(* Logix 5000 AddOnInstructionDefinition export Banner_K50ProTouch_Param_v4; software revision 33.00 *)

TYPE Banner_IOL_Port_v4 :   // UDT that has all of the data items necessary to communicate with a specific Port on a IO-Link Master
STRUCT
   Port_Controlled : INT;   // Each bit represents a port on an IO-Link Master. Set to 1 to tell AOI to control that port.
   Port_Activate : INT;   // Each bit represents a port on an IO-Link Master. When ON that port will process any commands in queue.
   Port_Read : INT;   // Each bit represents a port on an IO-Link Master. Used to determine when device AOI has requested a Read command.
   Port_Write : INT;   // Each bit represents a port on an IO-Link Master. Used to determine when device AOI has requested a Write command.
   Port_RW_Complete : INT;   // Each bit represents a port on an IO-Link Master. Tells device AOI that Read or Write request has been completed.
   Port_Device_Read : INT;
   Data_Transfer : SINT[190];   // Array to transfer data from IO-Master to device AOIs.
END_STRUCT
END_TYPE

TYPE Banner_K50ProTouch_RD_v4 :   // UDT with all of the Read only parameters for K50 Pro Touch.
STRUCT
   Master_Cycle_Time : INT;
   Min_Cycle_Time : INT;
   M_Sequence_Capability : INT;
   IO_Link_Version_ID : INT;
   Process_Data_Input_Length : INT;
   Process_Data_Output_Length : INT;
   Combined_Vendor_ID : DINT;   // IO-Link Vendor ID
   Vendor_ID1 : INT;
   Vendor_ID2 : INT;
   Combined_Device_ID : DINT;   // IO-Link Device ID
   Device_ID1 : INT;
   Device_ID2 : INT;
   Device_ID3 : INT;
   Serial_Number : STRING;
END_STRUCT
END_TYPE

TYPE Banner_K50ProTouch_SP_v4 :   // UDT for K50 Pro Touch with the State Parameters structure.
STRUCT
   Type : SINT;   // 0 = Off, 1 = Steady, 2 = Flash, 3 = Two Color Flash, 4 = 50/50, 5 = 50/50 Rotate, 6 = Chase, 7 = Intensity Sweep, 8 = Sequence.
   Direction : SINT;   // 0 = CCW, 1 = CW.
   Pattern : SINT;   // 0 = Flash, 1 = Strobe, 2 = Three Pulse, 3 = SOS, 4 = Random.
   Speed : SINT;   // 0 = Slow, 1 = Medium, 2 = Fast, 3 = Custom.
   Vibration_Feedback : SINT;   // 0 = Off, 1 = On, 2 = Pattern. Not available in all models.
   Off_Delay_Type : SINT;   // 0 =Leading Edge, 1 = Trailing Edge.
   Off_Delay : DINT;   // 0 to 65535 in ms. Length of time before the device returns to 'touch inactive' state after button is released.
   Static_Sequence : INT;   // 0 to 255. Value describing the LED position of the device.
   Sequence_Start_Location : SINT;   // 0 = LED1, 1 = LED2, 2 = LED3, 3 = LED4, 4 = LED5, 5 = LED6, 6 = LED7, 7 = LED8.
   Color_1 : SINT;   // 0 = Green, 1 = Red, 2 = Orange, 3 = Amber, 4 = Yellow, 5 = Lime Green, 6 = Spring Green, 7 = Cyan, 8 = SKy Blue, 9 = Blue, 10 = Violet, 11 = Magenta, 12 = Rose, 13 = White, 14 Custom 1, 15 = Custom 2.
   Color_1_Intensity : SINT;   // 0 = High, 1 = Medium, 2 = Low, 3 = Off, 4 = Custom.
   Color_2 : SINT;   // 0 = Green, 1 = Red, 2 = Orange, 3 = Amber, 4 = Yellow, 5 = Lime Green, 6 = Spring Green, 7 = Cyan, 8 = SKy Blue, 9 = Blue, 10 = Violet, 11 = Magenta, 12 = Rose, 13 = White, 14 Custom 1, 15 = Custom 2.
   Color_2_Intensity : SINT;   // 0 = High, 1 = Medium, 2 = Low, 3 = Off, 4 = Custom.
END_STRUCT
END_TYPE

TYPE Banner_K50ProTouch_v4 :   // UDT with all of the parameters for K50 Pro Touch.
STRUCT
   Initial_Global_Read : BOOL;   // Determines if all of the IO-Link data has been read into the PLC yet
   Command : INT;   // Value placed in here will activate a read or write to a specifc IO-Link Index
   Read_Data : Banner_K50ProTouch_RD_v4;   // All read data
   Write_Data : Banner_K50ProTouch_WD_v4;   // All data that can be written to.
   Archive : Banner_K50ProTouch_WD_v4;   // Archive of the write data.
   Reset : BOOL;
END_STRUCT
END_TYPE

TYPE Banner_K50ProTouch_WD_v4 :   // UDT that stores the Write Data for a K50 Pro Touch.
STRUCT
   System_Command : INT;   // See IODD file for list of commands that can be activated via the System Command interface
   Parameter_Access_Lock : SINT;   // Write access to all read/write parameters is block when this bit is ON.
   Data_Storage_Lock : SINT;   // Data storage mechanism is inhibited when bit is ON.
   Local_Parameterization_Lock : SINT;   // Parameteriation via local control elementes is inhibited.
   Local_User_Interface_Lock : SINT;   // Operation of the hmi on the device is disabled.
   Operation_Mode : SINT;   // 0 = Multicolor, 1 = Four State Full Logic, 2 = Advanced, 3 = LED Control, 4 = Demo.
   Custom_Intensity : SINT;   // 0 to 100 %
   Custom_Flash_Rate : INT;   // Range 5 to 200 (.5 to 20 converted rate).
   Restrict_to_Gamut : SINT;   // 0 = Off, 1 = On.
   Touch_Sensitivity : SINT;   // 0 = Low, 1 = High.
   Function : SINT;   // 0 = Momentary, 1 = Latched.
   Mute_Enable : SINT;   // 0 = Off, 1 = On.
   On_Delay : DINT;   // 0 to 65535 in ms. Length of time the touch button needs to be pressed to trigger touch active state.
   Output_State : SINT;   // 0 = NO, 1 = NC.
   Off_Delay_Type : SINT;   // 0 = Leading Edge, 1 = Trailing Edge.
   Off_Delay : DINT;   // 0 to 65535 in ms. Length of time before the device returns to the 'touch inactive' state after button is released.
   State_Parameters : Banner_K50ProTouch_SP_v4[5];   // State Parameters. 1 through 4 will have values.
   CC1_Red : INT;   // 0-255. Custom 1 Red.
   CC1_Green : INT;   // 0-255. Custom 1 Green.
   CC1_Blue : INT;   // 0-255. Custom 1 Blue.
   CC2_Red : INT;   // 0-255. Custom 2 Red.
   CC2_Green : INT;   // 0-255. Custom 2 Green.
   CC_Blue : INT;   // 0-255. Custom 2 Blue.
END_STRUCT
END_TYPE

ADD_ON_INSTRUCTION Banner_K50ProTouch_Param_v4   (* revision 4.2, vendor Banner Engineering *)
// AOI to read and write parameter data to an IO-Link K50 Pro Touch.
// Revision note:
// Write operation for Index 82 and 83 had wrong size. Changed szie to value of 3.
VAR_IN_OUT
   K50ProTouch : Banner_K50ProTouch_v4; {required}
   Port_Data : Banner_IOL_Port_v4; {required}
END_VAR
VAR_INPUT
   Port : DINT; {required}
END_VAR
VAR
   Local_Control : DINT; {access None}
   Global_Read_Command_Value : INT; {access None}
   Global_Write_Command_Value : INT; {access None}
   Command_Being_Processed : BOOL; {access None}
   Update_Archive : BOOL; {access None}
   Index_Write_Control : DINT; {access None}
   Index_Write_Inprocess : INT; {access None}
   Temp_Excess_Gain : DINT[2]; {access None}
   Inprocess_Index : DINT; {access None}
   SP_Index : DINT; {access None}   // State Parameters Index
   SP_Write_Index : DINT; {access None}
   SP_R_Index : DINT; {access None}
   SP_W_Index : DINT; {access None}
END_VAR

ROUTINE Logic   (* ladder *)
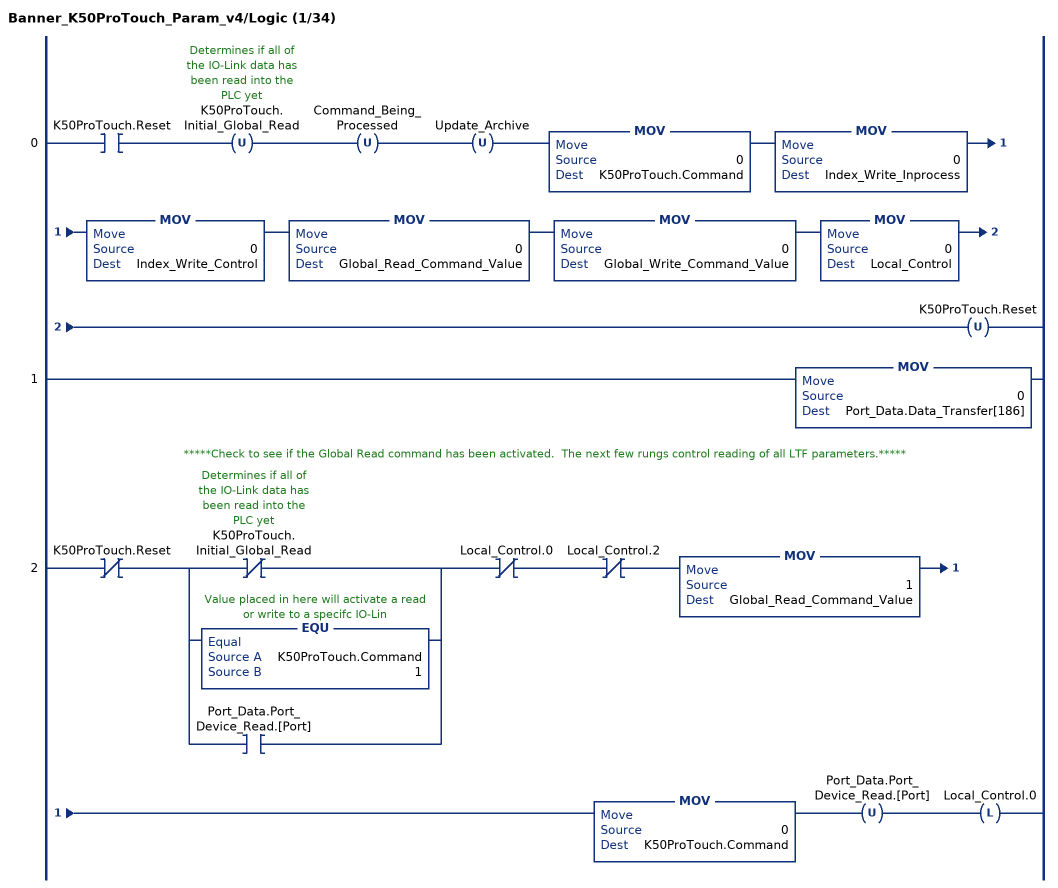
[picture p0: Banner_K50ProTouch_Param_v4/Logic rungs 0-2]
   0: XIC(K50ProTouch.Reset)OTU(K50ProTouch.Initial_Global_Read)OTU(Command_Being_Processed)OTU(Update_Archive)MOV(0,K50ProTouch.Command)MOV(0,Index_Write_Inprocess)MOV(0,Index_Write_Control)MOV(0,Global_Read_Command_Value)MOV(0,Global_Write_Command_Value)MOV(0,Local_Control)OTU(K50ProTouch.Reset);
   1: MOV(0,Port_Data.Data_Transfer[186]);
   // *****Check to see if the Global Read command has been activated.  The next few rungs control reading of all LTF parameters.*****
   2: XIO(K50ProTouch.Reset)[XIO(K50ProTouch.Initial_Global_Read) ,EQU(K50ProTouch.Command,1) ,XIC(Port_Data.Port_Device_Read.[Port]) ]XIO(Local_Control.0)XIO(Local_Control.2)MOV(1,Global_Read_Command_Value)MOV(0,K50ProTouch.Command)OTU(Port_Data.Port_Device_Read.[Port])OTL(Local_Control.0);
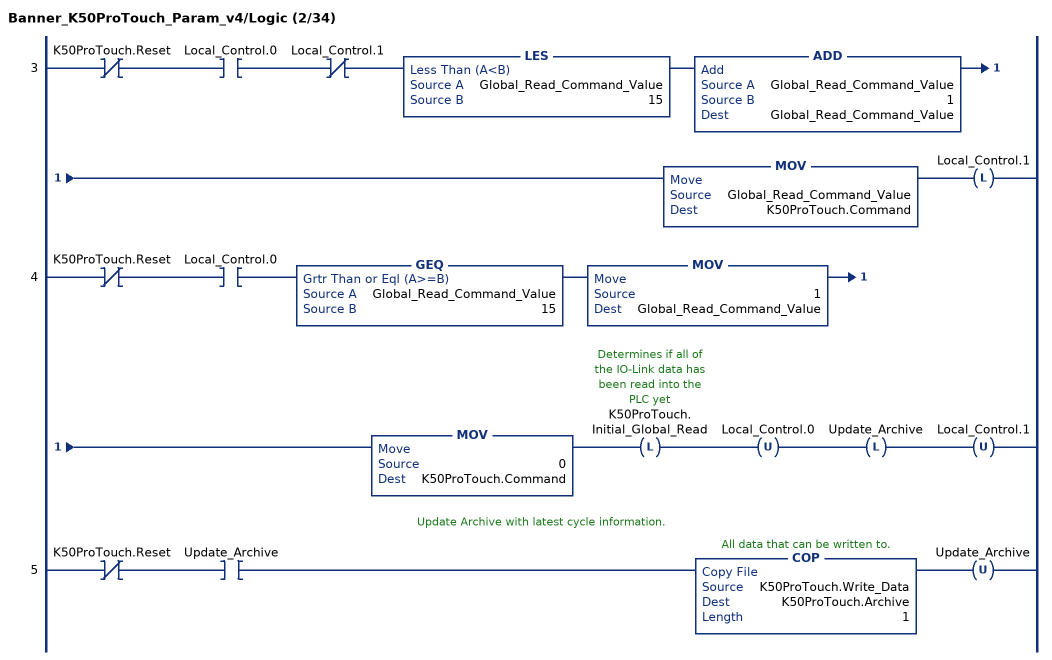
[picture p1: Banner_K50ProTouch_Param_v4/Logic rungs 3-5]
   3: XIO(K50ProTouch.Reset)XIC(Local_Control.0)XIO(Local_Control.1)LES(Global_Read_Command_Value,15)ADD(Global_Read_Command_Value,1,Global_Read_Command_Value)MOV(Global_Read_Command_Value,K50ProTouch.Command)OTL(Local_Control.1);
   4: XIO(K50ProTouch.Reset)XIC(Local_Control.0)GEQ(Global_Read_Command_Value,15)MOV(1,Global_Read_Command_Value)MOV(0,K50ProTouch.Command)OTL(K50ProTouch.Initial_Global_Read)OTU(Local_Control.0)OTL(Update_Archive)OTU(Local_Control.1);
   // Update Archive with latest cycle information.
   5: XIO(K50ProTouch.Reset)XIC(Update_Archive)COP(K50ProTouch.Write_Data,K50ProTouch.Archive,1)OTU(Update_Archive);
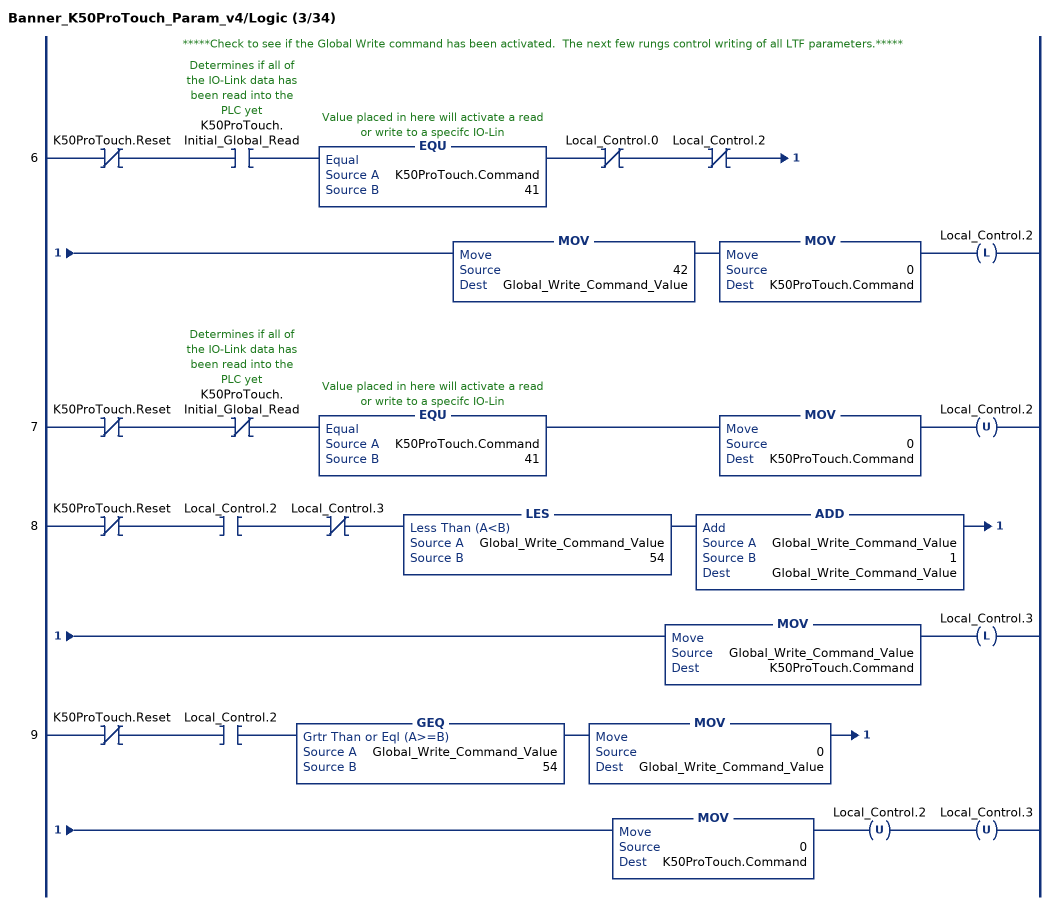
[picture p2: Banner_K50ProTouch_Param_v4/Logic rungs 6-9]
   // *****Check to see if the Global Write command has been activated.  The next few rungs control writing of all LTF parameters.*****
   6: XIO(K50ProTouch.Reset)XIC(K50ProTouch.Initial_Global_Read)EQU(K50ProTouch.Command,41)XIO(Local_Control.0)XIO(Local_Control.2)MOV(42,Global_Write_Command_Value)MOV(0,K50ProTouch.Command)OTL(Local_Control.2);
   7: XIO(K50ProTouch.Reset)XIO(K50ProTouch.Initial_Global_Read)EQU(K50ProTouch.Command,41)MOV(0,K50ProTouch.Command)OTU(Local_Control.2);
   8: XIO(K50ProTouch.Reset)XIC(Local_Control.2)XIO(Local_Control.3)LES(Global_Write_Command_Value,54)ADD(Global_Write_Command_Value,1,Global_Write_Command_Value)MOV(Global_Write_Command_Value,K50ProTouch.Command)OTL(Local_Control.3);
   9: XIO(K50ProTouch.Reset)XIC(Local_Control.2)GEQ(Global_Write_Command_Value,54)MOV(0,Global_Write_Command_Value)MOV(0,K50ProTouch.Command)OTU(Local_Control.2)OTU(Local_Control.3);
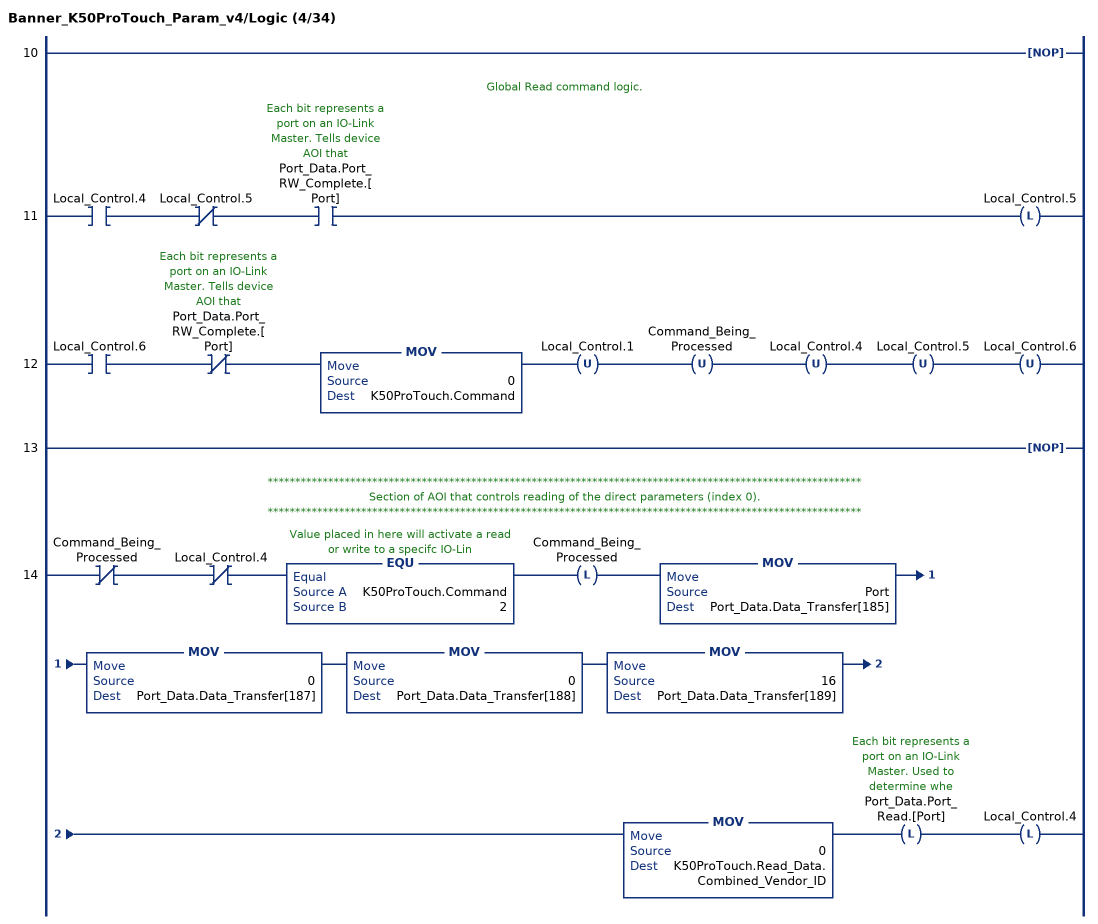
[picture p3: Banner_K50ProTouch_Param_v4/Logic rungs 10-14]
   10: NOP();
   // Global Read command logic.
   11: XIC(Local_Control.4)XIO(Local_Control.5)XIC(Port_Data.Port_RW_Complete.[Port])OTL(Local_Control.5);
   12: XIC(Local_Control.6)XIO(Port_Data.Port_RW_Complete.[Port])MOV(0,K50ProTouch.Command)OTU(Local_Control.1)OTU(Command_Being_Processed)OTU(Local_Control.4)OTU(Local_Control.5)OTU(Local_Control.6);
   13: NOP();
   // ************************************************************************************************************
   // Section of AOI that controls reading of the direct parameters (index 0).
   // ************************************************************************************************************
   14: XIO(Command_Being_Processed)XIO(Local_Control.4)EQU(K50ProTouch.Command,2)OTL(Command_Being_Processed)MOV(Port,Port_Data.Data_Transfer[185])MOV(0,Port_Data.Data_Transfer[187])MOV(0,Port_Data.Data_Transfer[188])MOV(16,Port_Data.Data_Transfer[189])MOV(0,K50ProTouch.Read_Data.Combined_Vendor_ID)OTL(Port_Data.Port_Read.[Port])OTL(Local_Control.4);
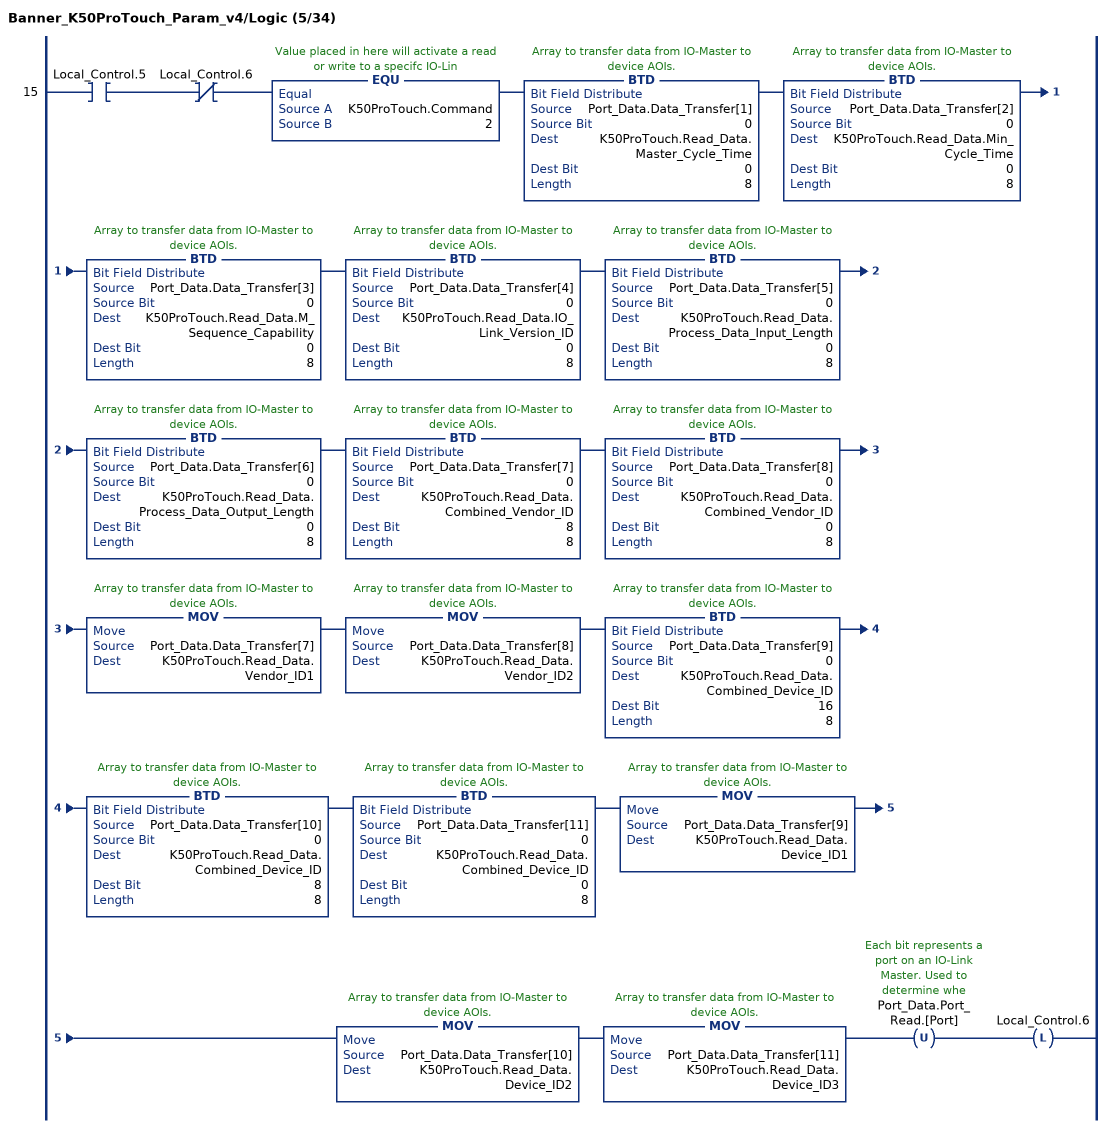
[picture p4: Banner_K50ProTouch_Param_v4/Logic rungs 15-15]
   15: XIC(Local_Control.5)XIO(Local_Control.6)EQU(K50ProTouch.Command,2)BTD(Port_Data.Data_Transfer[1],0,K50ProTouch.Read_Data.Master_Cycle_Time,0,8)BTD(Port_Data.Data_Transfer[2],0,K50ProTouch.Read_Data.Min_Cycle_Time,0,8)BTD(Port_Data.Data_Transfer[3],0,K50ProTouch.Read_Data.M_Sequence_Capability,0,8)BTD(Port_Data.Data_Transfer[4],0,K50ProTouch.Read_Data.IO_Link_Version_ID,0,8)BTD(Port_Data.Data_Transfer[5],0,K50ProTouch.Read_Data.Process_Data_Input_Length,0,8)BTD(Port_Data.Data_Transfer[6],0,K50ProTouch.Read_Data.Process_Data_Output_Length,0,8)BTD(Port_Data.Data_Transfer[7],0,K50ProTouch.Read_Data.Combined_Vendor_ID,8,8)BTD(Port_Data.Data_Transfer[8],0,K50ProTouch.Read_Data.Combined_Vendor_ID,0,8)MOV(Port_Data.Data_Transfer[7],K50ProTouch.Read_Data.Vendor_ID1)MOV(Port_Data.Data_Transfer[8],K50ProTouch.Read_Data.Vendor_ID2)BTD(Port_Data.Data_Transfer[9],0,K50ProTouch.Read_Data.Combined_Device_ID,16,8)BTD(Port_Data.Data_Transfer[10],0,K50ProTouch.Read_Data.Combined_Device_ID,8,8)BTD(Port_Data.Data_Transfer[11],0,K50ProTouch.Read_Data.Combined_Device_ID,0,8)MOV(Port_Data.Data_Transfer[9],K50ProTouch.Read_Data.Device_ID1)MOV(Port_Data.Data_Transfer[10],K50ProTouch.Read_Data.Device_ID2)MOV(Port_Data.Data_Transfer[11],K50ProTouch.Read_Data.Device_ID3)OTU(Port_Data.Port_Read.[Port])OTL(Local_Control.6);
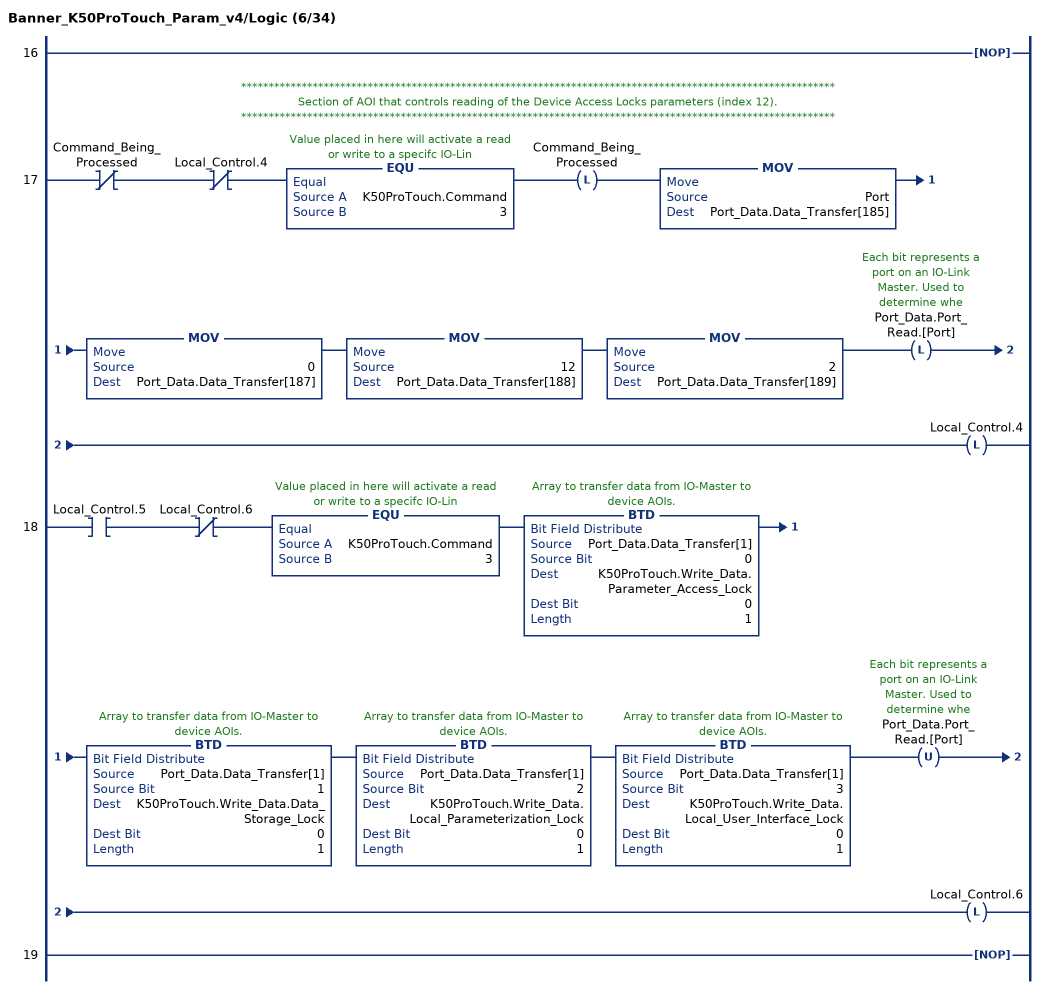
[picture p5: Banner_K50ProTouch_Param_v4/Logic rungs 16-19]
   16: NOP();
   // ************************************************************************************************************
   // Section of AOI that controls reading of the Device Access Locks parameters (index 12).
   // ************************************************************************************************************
   17: XIO(Command_Being_Processed)XIO(Local_Control.4)EQU(K50ProTouch.Command,3)OTL(Command_Being_Processed)MOV(Port,Port_Data.Data_Transfer[185])MOV(0,Port_Data.Data_Transfer[187])MOV(12,Port_Data.Data_Transfer[188])MOV(2,Port_Data.Data_Transfer[189])OTL(Port_Data.Port_Read.[Port])OTL(Local_Control.4);
   18: XIC(Local_Control.5)XIO(Local_Control.6)EQU(K50ProTouch.Command,3)BTD(Port_Data.Data_Transfer[1],0,K50ProTouch.Write_Data.Parameter_Access_Lock,0,1)BTD(Port_Data.Data_Transfer[1],1,K50ProTouch.Write_Data.Data_Storage_Lock,0,1)BTD(Port_Data.Data_Transfer[1],2,K50ProTouch.Write_Data.Local_Parameterization_Lock,0,1)BTD(Port_Data.Data_Transfer[1],3,K50ProTouch.Write_Data.Local_User_Interface_Lock,0,1)OTU(Port_Data.Port_Read.[Port])OTL(Local_Control.6);
   19: NOP();
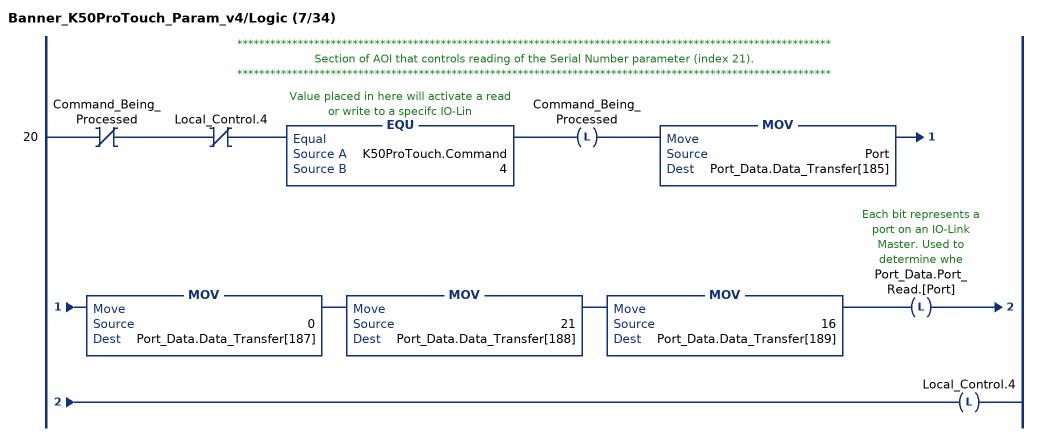
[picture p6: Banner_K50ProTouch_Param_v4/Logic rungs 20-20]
   // ************************************************************************************************************
   // Section of AOI that controls reading of the Serial Number parameter (index 21).
   // ************************************************************************************************************
   20: XIO(Command_Being_Processed)XIO(Local_Control.4)EQU(K50ProTouch.Command,4)OTL(Command_Being_Processed)MOV(Port,Port_Data.Data_Transfer[185])MOV(0,Port_Data.Data_Transfer[187])MOV(21,Port_Data.Data_Transfer[188])MOV(16,Port_Data.Data_Transfer[189])OTL(Port_Data.Port_Read.[Port])OTL(Local_Control.4);
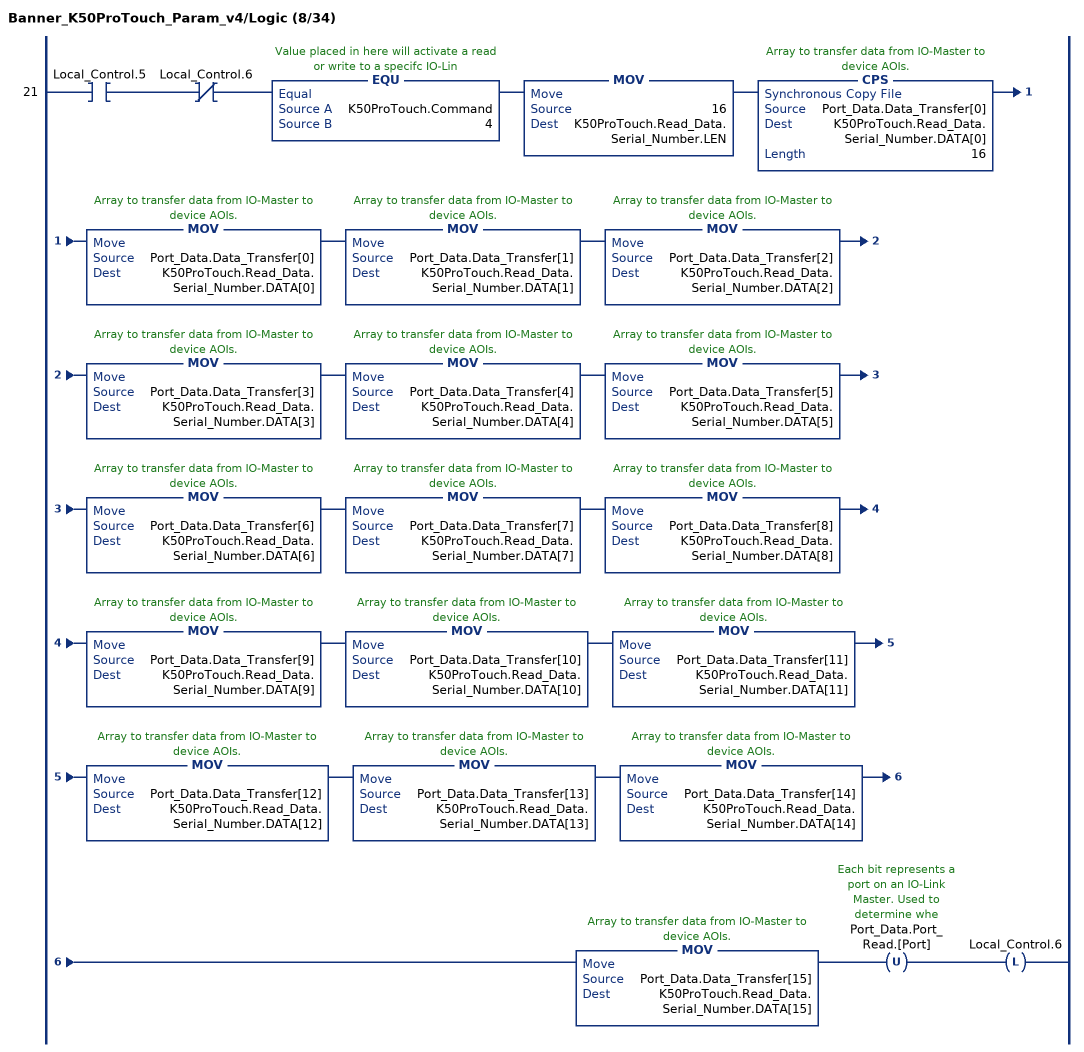
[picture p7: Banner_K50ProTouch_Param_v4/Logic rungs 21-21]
   21: XIC(Local_Control.5)XIO(Local_Control.6)EQU(K50ProTouch.Command,4)MOV(16,K50ProTouch.Read_Data.Serial_Number.LEN)CPS(Port_Data.Data_Transfer[0],K50ProTouch.Read_Data.Serial_Number.DATA[0],16)MOV(Port_Data.Data_Transfer[0],K50ProTouch.Read_Data.Serial_Number.DATA[0])MOV(Port_Data.Data_Transfer[1],K50ProTouch.Read_Data.Serial_Number.DATA[1])MOV(Port_Data.Data_Transfer[2],K50ProTouch.Read_Data.Serial_Number.DATA[2])MOV(Port_Data.Data_Transfer[3],K50ProTouch.Read_Data.Serial_Number.DATA[3])MOV(Port_Data.Data_Transfer[4],K50ProTouch.Read_Data.Serial_Number.DATA[4])MOV(Port_Data.Data_Transfer[5],K50ProTouch.Read_Data.Serial_Number.DATA[5])MOV(Port_Data.Data_Transfer[6],K50ProTouch.Read_Data.Serial_Number.DATA[6])MOV(Port_Data.Data_Transfer[7],K50ProTouch.Read_Data.Serial_Number.DATA[7])MOV(Port_Data.Data_Transfer[8],K50ProTouch.Read_Data.Serial_Number.DATA[8])MOV(Port_Data.Data_Transfer[9],K50ProTouch.Read_Data.Serial_Number.DATA[9])MOV(Port_Data.Data_Transfer[10],K50ProTouch.Read_Data.Serial_Number.DATA[10])MOV(Port_Data.Data_Transfer[11],K50ProTouch.Read_Data.Serial_Number.DATA[11])MOV(Port_Data.Data_Transfer[12],K50ProTouch.Read_Data.Serial_Number.DATA[12])MOV(Port_Data.Data_Transfer[13],K50ProTouch.Read_Data.Serial_Number.DATA[13])MOV(Port_Data.Data_Transfer[14],K50ProTouch.Read_Data.Serial_Number.DATA[14])MOV(Port_Data.Data_Transfer[15],K50ProTouch.Read_Data.Serial_Number.DATA[15])OTU(Port_Data.Port_Read.[Port])OTL(Local_Control.6);
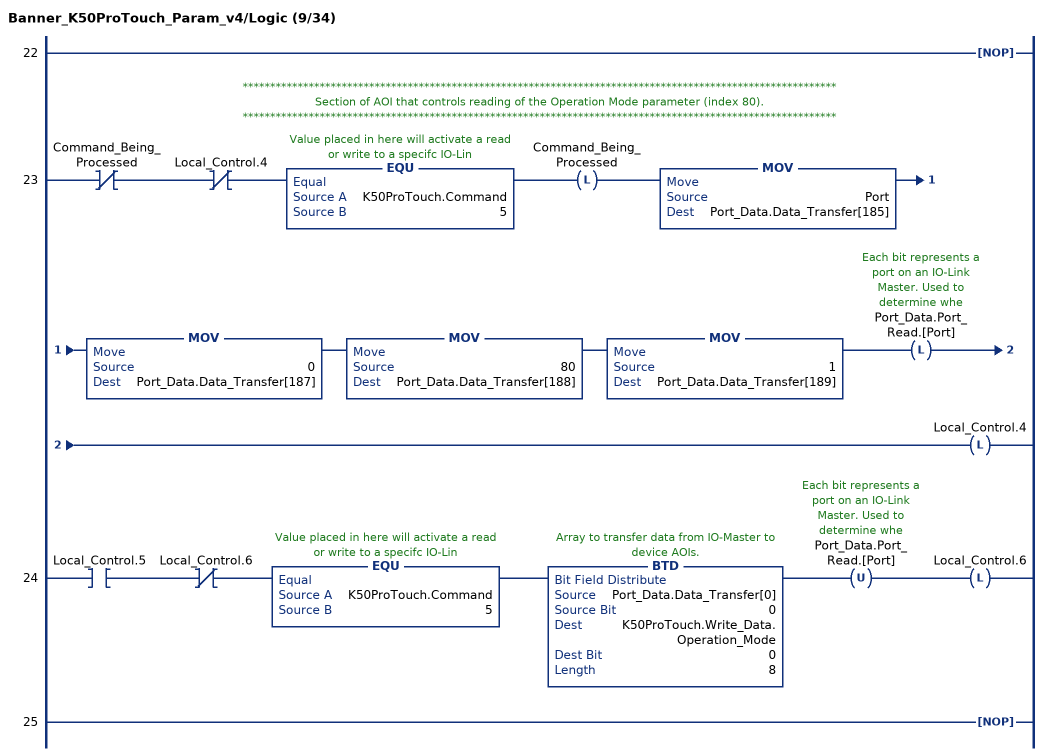
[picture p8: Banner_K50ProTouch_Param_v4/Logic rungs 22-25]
   22: NOP();
   // ************************************************************************************************************
   // Section of AOI that controls reading of the Operation Mode parameter (index 80).
   // ************************************************************************************************************
   23: XIO(Command_Being_Processed)XIO(Local_Control.4)EQU(K50ProTouch.Command,5)OTL(Command_Being_Processed)MOV(Port,Port_Data.Data_Transfer[185])MOV(0,Port_Data.Data_Transfer[187])MOV(80,Port_Data.Data_Transfer[188])MOV(1,Port_Data.Data_Transfer[189])OTL(Port_Data.Port_Read.[Port])OTL(Local_Control.4);
   24: XIC(Local_Control.5)XIO(Local_Control.6)EQU(K50ProTouch.Command,5)BTD(Port_Data.Data_Transfer[0],0,K50ProTouch.Write_Data.Operation_Mode,0,8)OTU(Port_Data.Port_Read.[Port])OTL(Local_Control.6);
   25: NOP();
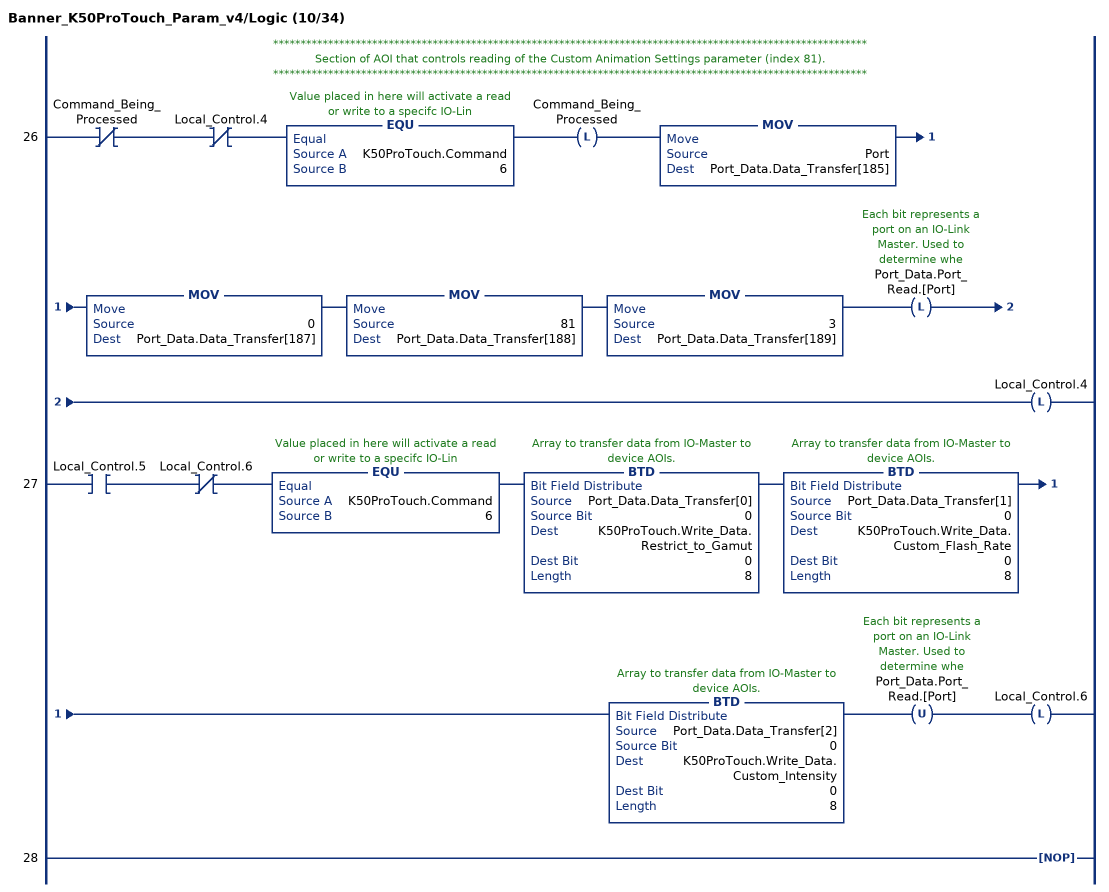
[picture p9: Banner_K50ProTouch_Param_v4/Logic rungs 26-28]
   // ************************************************************************************************************
   // Section of AOI that controls reading of the Custom Animation Settings parameter (index 81).
   // ************************************************************************************************************
   26: XIO(Command_Being_Processed)XIO(Local_Control.4)EQU(K50ProTouch.Command,6)OTL(Command_Being_Processed)MOV(Port,Port_Data.Data_Transfer[185])MOV(0,Port_Data.Data_Transfer[187])MOV(81,Port_Data.Data_Transfer[188])MOV(3,Port_Data.Data_Transfer[189])OTL(Port_Data.Port_Read.[Port])OTL(Local_Control.4);
   27: XIC(Local_Control.5)XIO(Local_Control.6)EQU(K50ProTouch.Command,6)BTD(Port_Data.Data_Transfer[0],0,K50ProTouch.Write_Data.Restrict_to_Gamut,0,8)BTD(Port_Data.Data_Transfer[1],0,K50ProTouch.Write_Data.Custom_Flash_Rate,0,8)BTD(Port_Data.Data_Transfer[2],0,K50ProTouch.Write_Data.Custom_Intensity,0,8)OTU(Port_Data.Port_Read.[Port])OTL(Local_Control.6);
   28: NOP();
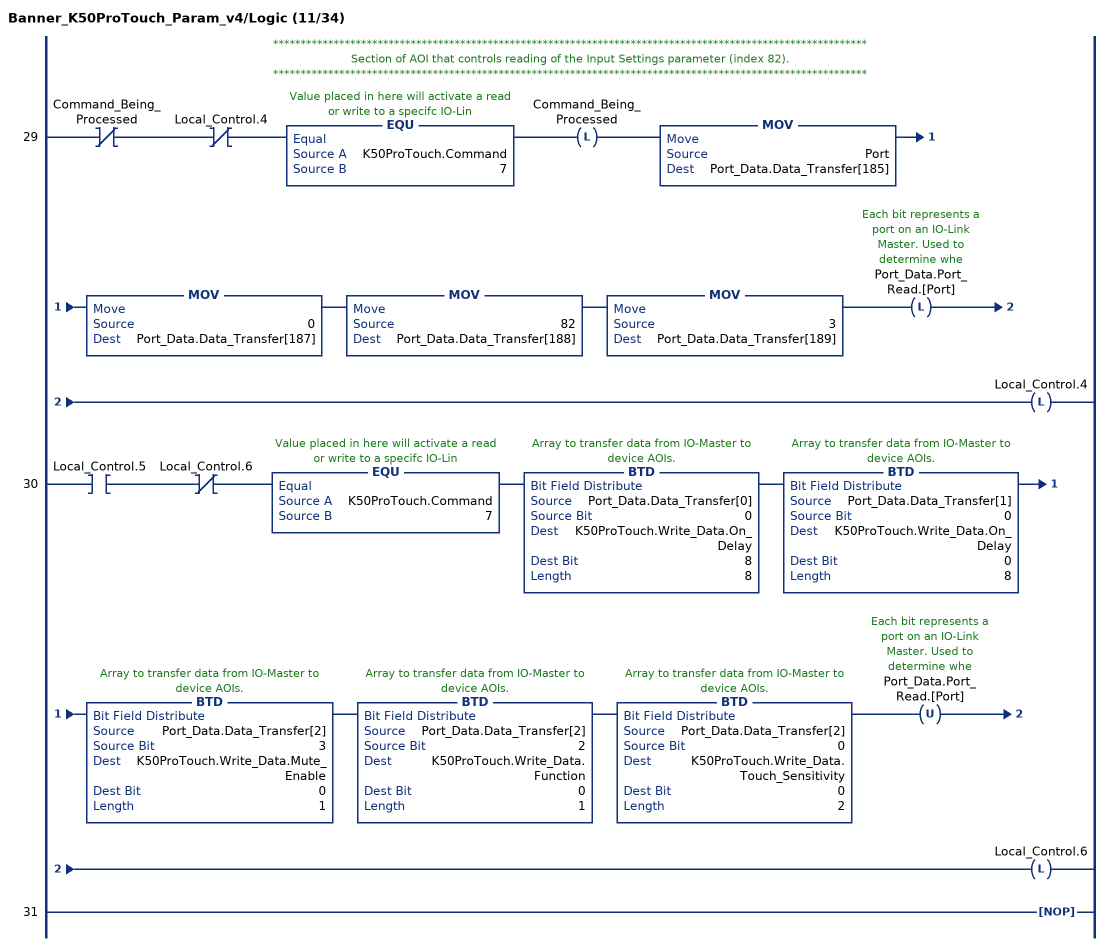
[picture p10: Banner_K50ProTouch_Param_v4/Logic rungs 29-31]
   // ************************************************************************************************************
   // Section of AOI that controls reading of the Input Settings parameter (index 82).
   // ************************************************************************************************************
   29: XIO(Command_Being_Processed)XIO(Local_Control.4)EQU(K50ProTouch.Command,7)OTL(Command_Being_Processed)MOV(Port,Port_Data.Data_Transfer[185])MOV(0,Port_Data.Data_Transfer[187])MOV(82,Port_Data.Data_Transfer[188])MOV(3,Port_Data.Data_Transfer[189])OTL(Port_Data.Port_Read.[Port])OTL(Local_Control.4);
   30: XIC(Local_Control.5)XIO(Local_Control.6)EQU(K50ProTouch.Command,7)BTD(Port_Data.Data_Transfer[0],0,K50ProTouch.Write_Data.On_Delay,8,8)BTD(Port_Data.Data_Transfer[1],0,K50ProTouch.Write_Data.On_Delay,0,8)BTD(Port_Data.Data_Transfer[2],3,K50ProTouch.Write_Data.Mute_Enable,0,1)BTD(Port_Data.Data_Transfer[2],2,K50ProTouch.Write_Data.Function,0,1)BTD(Port_Data.Data_Transfer[2],0,K50ProTouch.Write_Data.Touch_Sensitivity,0,2)OTU(Port_Data.Port_Read.[Port])OTL(Local_Control.6);
   31: NOP();
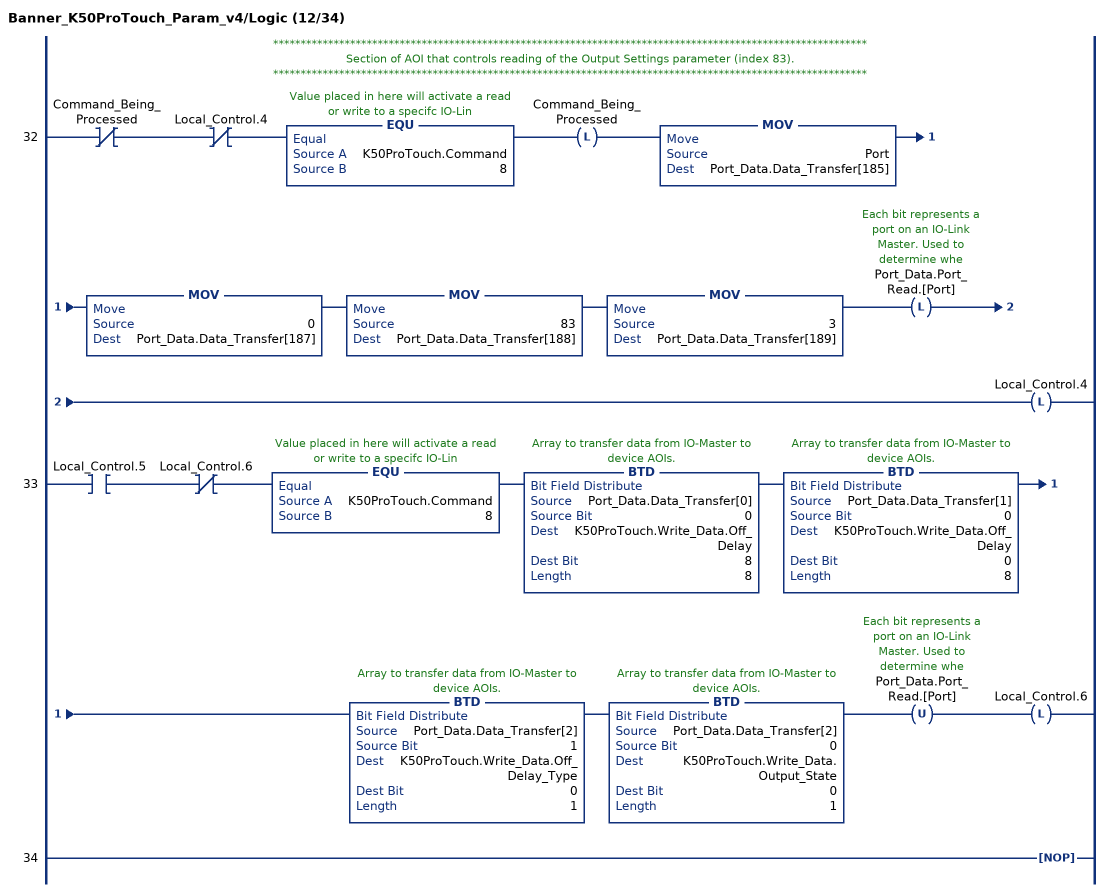
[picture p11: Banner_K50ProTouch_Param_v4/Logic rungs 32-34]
   // ************************************************************************************************************
   // Section of AOI that controls reading of the Output Settings parameter (index 83).
   // ************************************************************************************************************
   32: XIO(Command_Being_Processed)XIO(Local_Control.4)EQU(K50ProTouch.Command,8)OTL(Command_Being_Processed)MOV(Port,Port_Data.Data_Transfer[185])MOV(0,Port_Data.Data_Transfer[187])MOV(83,Port_Data.Data_Transfer[188])MOV(3,Port_Data.Data_Transfer[189])OTL(Port_Data.Port_Read.[Port])OTL(Local_Control.4);
   33: XIC(Local_Control.5)XIO(Local_Control.6)EQU(K50ProTouch.Command,8)BTD(Port_Data.Data_Transfer[0],0,K50ProTouch.Write_Data.Off_Delay,8,8)BTD(Port_Data.Data_Transfer[1],0,K50ProTouch.Write_Data.Off_Delay,0,8)BTD(Port_Data.Data_Transfer[2],1,K50ProTouch.Write_Data.Off_Delay_Type,0,1)BTD(Port_Data.Data_Transfer[2],0,K50ProTouch.Write_Data.Output_State,0,1)OTU(Port_Data.Port_Read.[Port])OTL(Local_Control.6);
   34: NOP();
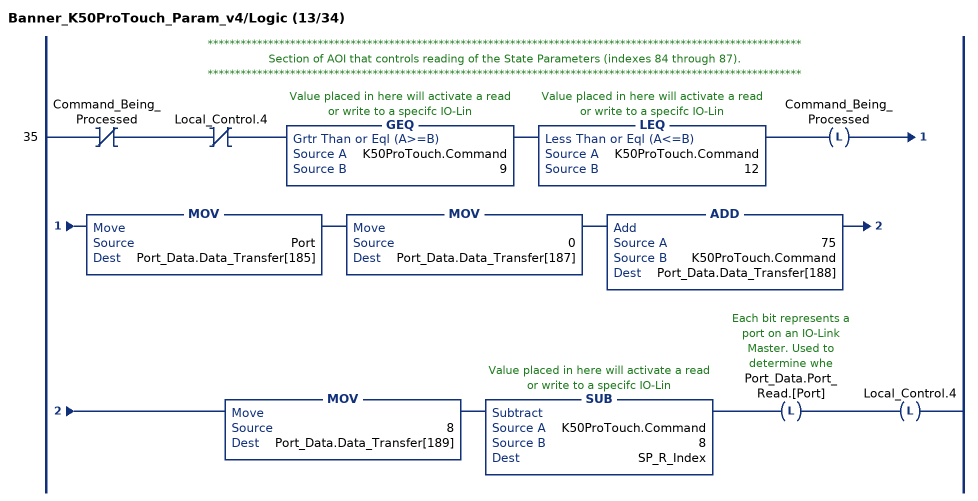
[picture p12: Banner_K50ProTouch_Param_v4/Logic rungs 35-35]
   // ************************************************************************************************************
   // Section of AOI that controls reading of the State Parameters (indexes 84 through 87).
   // ************************************************************************************************************
   35: XIO(Command_Being_Processed)XIO(Local_Control.4)GEQ(K50ProTouch.Command,9)LEQ(K50ProTouch.Command,12)OTL(Command_Being_Processed)MOV(Port,Port_Data.Data_Transfer[185])MOV(0,Port_Data.Data_Transfer[187])ADD(75,K50ProTouch.Command,Port_Data.Data_Transfer[188])MOV(8,Port_Data.Data_Transfer[189])SUB(K50ProTouch.Command,8,SP_R_Index)OTL(Port_Data.Port_Read.[Port])OTL(Local_Control.4);
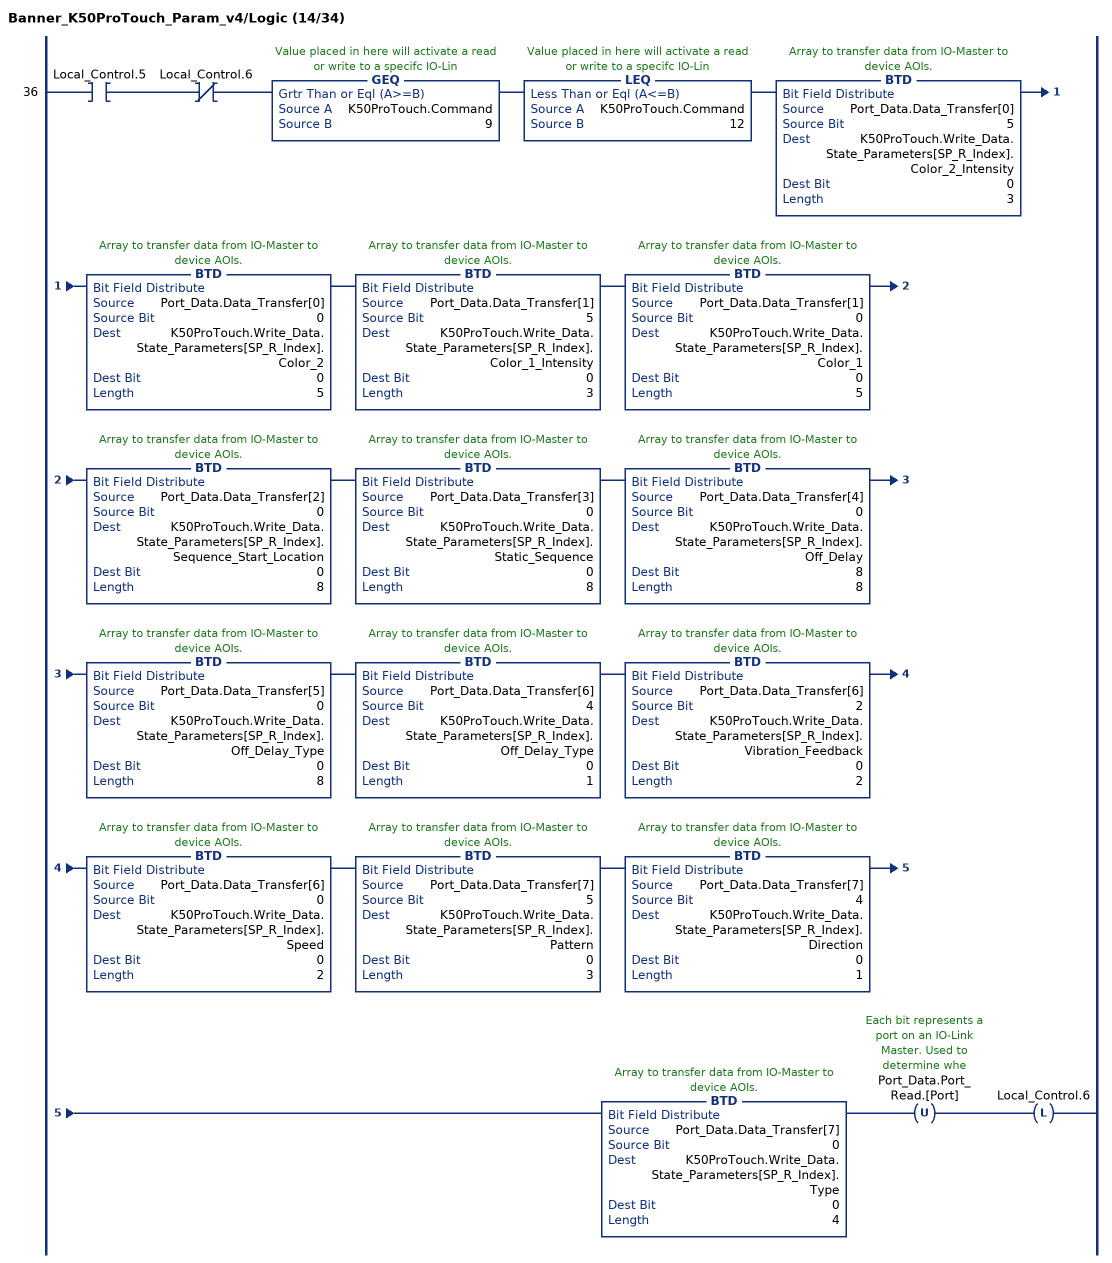
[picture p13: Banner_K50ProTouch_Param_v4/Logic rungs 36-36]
   36: XIC(Local_Control.5)XIO(Local_Control.6)GEQ(K50ProTouch.Command,9)LEQ(K50ProTouch.Command,12)BTD(Port_Data.Data_Transfer[0],5,K50ProTouch.Write_Data.State_Parameters[SP_R_Index].Color_2_Intensity,0,3)BTD(Port_Data.Data_Transfer[0],0,K50ProTouch.Write_Data.State_Parameters[SP_R_Index].Color_2,0,5)BTD(Port_Data.Data_Transfer[1],5,K50ProTouch.Write_Data.State_Parameters[SP_R_Index].Color_1_Intensity,0,3)BTD(Port_Data.Data_Transfer[1],0,K50ProTouch.Write_Data.State_Parameters[SP_R_Index].Color_1,0,5)BTD(Port_Data.Data_Transfer[2],0,K50ProTouch.Write_Data.State_Parameters[SP_R_Index].Sequence_Start_Location,0,8)BTD(Port_Data.Data_Transfer[3],0,K50ProTouch.Write_Data.State_Parameters[SP_R_Index].Static_Sequence,0,8)BTD(Port_Data.Data_Transfer[4],0,K50ProTouch.Write_Data.State_Parameters[SP_R_Index].Off_Delay,8,8)BTD(Port_Data.Data_Transfer[5],0,K50ProTouch.Write_Data.State_Parameters[SP_R_Index].Off_Delay_Type,0,8)BTD(Port_Data.Data_Transfer[6],4,K50ProTouch.Write_Data.State_Parameters[SP_R_Index].Off_Delay_Type,0,1)BTD(Port_Data.Data_Transfer[6],2,K50ProTouch.Write_Data.State_Parameters[SP_R_Index].Vibration_Feedback,0,2)BTD(Port_Data.Data_Transfer[6],0,K50ProTouch.Write_Data.State_Parameters[SP_R_Index].Speed,0,2)BTD(Port_Data.Data_Transfer[7],5,K50ProTouch.Write_Data.State_Parameters[SP_R_Index].Pattern,0,3)BTD(Port_Data.Data_Transfer[7],4,K50ProTouch.Write_Data.State_Parameters[SP_R_Index].Direction,0,1)BTD(Port_Data.Data_Transfer[7],0,K50ProTouch.Write_Data.State_Parameters[SP_R_Index].Type,0,4)OTU(Port_Data.Port_Read.[Port])OTL(Local_Control.6);
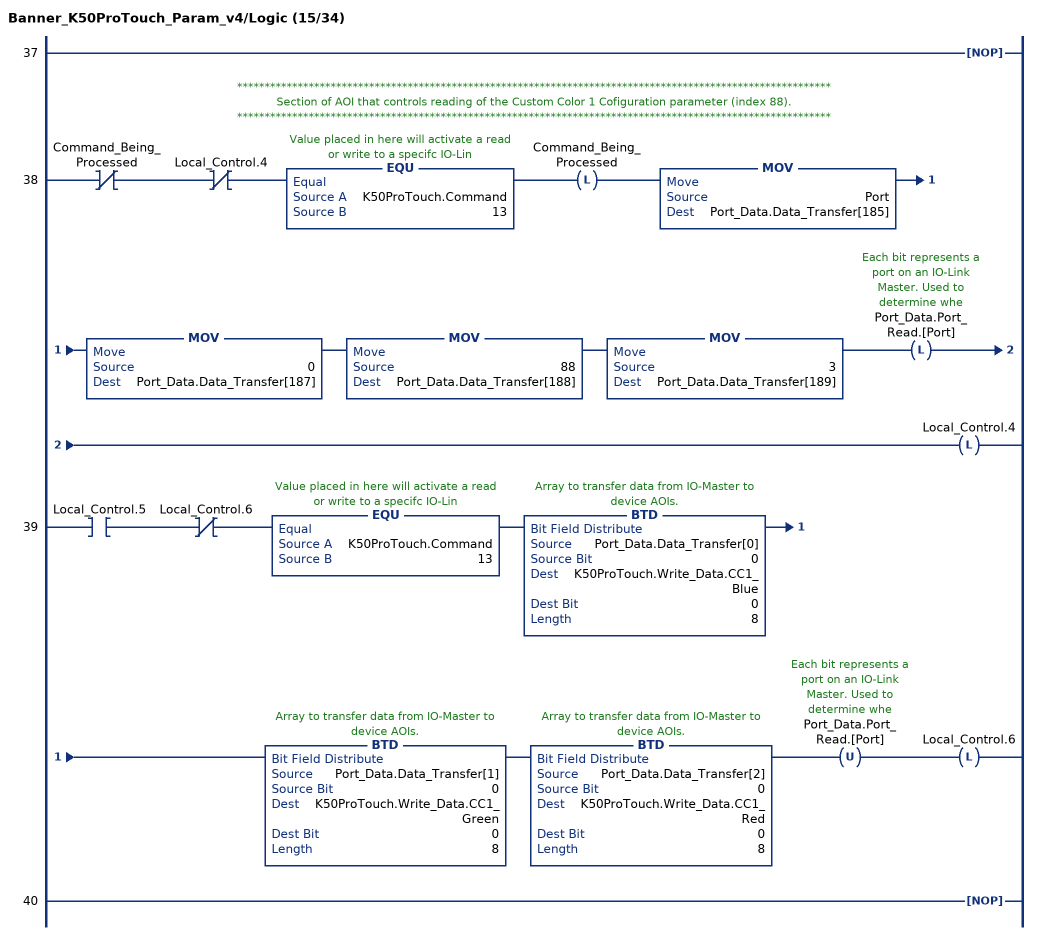
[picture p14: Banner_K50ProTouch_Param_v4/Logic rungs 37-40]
   37: NOP();
   // ************************************************************************************************************
   // Section of AOI that controls reading of the Custom Color 1 Cofiguration parameter (index 88).
   // ************************************************************************************************************
   38: XIO(Command_Being_Processed)XIO(Local_Control.4)EQU(K50ProTouch.Command,13)OTL(Command_Being_Processed)MOV(Port,Port_Data.Data_Transfer[185])MOV(0,Port_Data.Data_Transfer[187])MOV(88,Port_Data.Data_Transfer[188])MOV(3,Port_Data.Data_Transfer[189])OTL(Port_Data.Port_Read.[Port])OTL(Local_Control.4);
   39: XIC(Local_Control.5)XIO(Local_Control.6)EQU(K50ProTouch.Command,13)BTD(Port_Data.Data_Transfer[0],0,K50ProTouch.Write_Data.CC1_Blue,0,8)BTD(Port_Data.Data_Transfer[1],0,K50ProTouch.Write_Data.CC1_Green,0,8)BTD(Port_Data.Data_Transfer[2],0,K50ProTouch.Write_Data.CC1_Red,0,8)OTU(Port_Data.Port_Read.[Port])OTL(Local_Control.6);
   40: NOP();
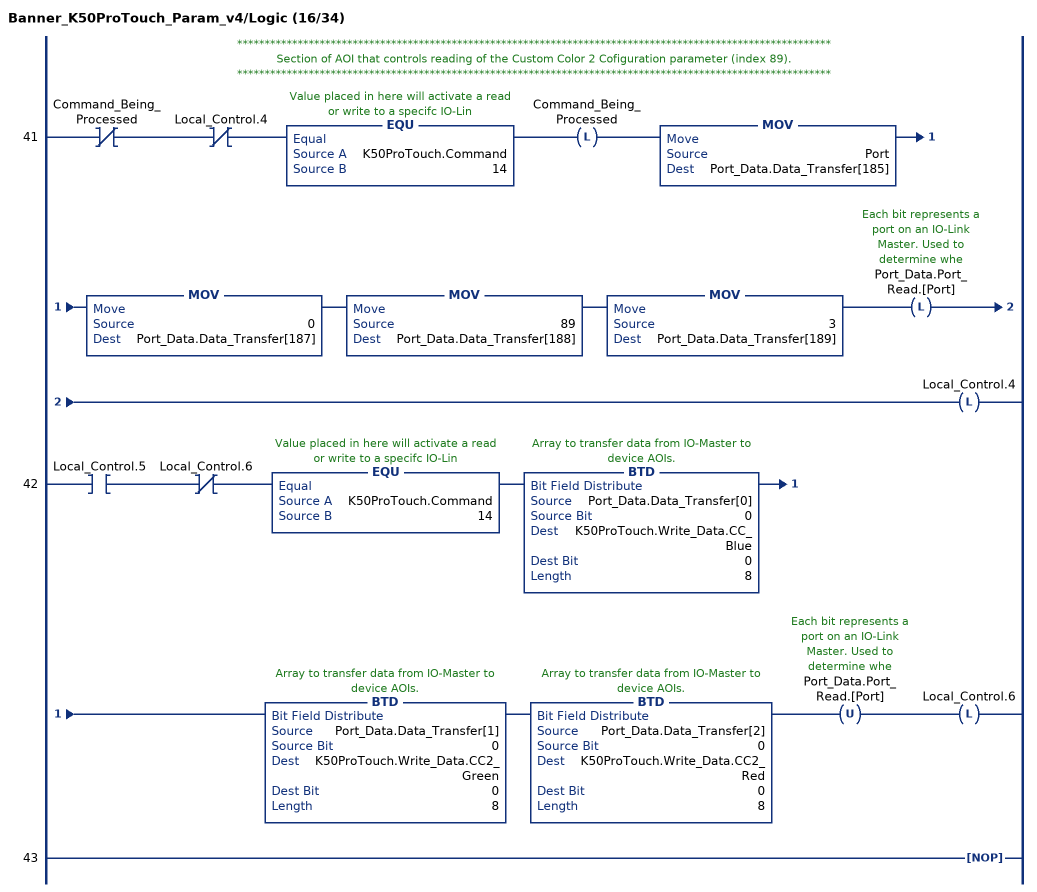
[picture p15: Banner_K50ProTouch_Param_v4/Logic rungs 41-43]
   // ************************************************************************************************************
   // Section of AOI that controls reading of the Custom Color 2 Cofiguration parameter (index 89).
   // ************************************************************************************************************
   41: XIO(Command_Being_Processed)XIO(Local_Control.4)EQU(K50ProTouch.Command,14)OTL(Command_Being_Processed)MOV(Port,Port_Data.Data_Transfer[185])MOV(0,Port_Data.Data_Transfer[187])MOV(89,Port_Data.Data_Transfer[188])MOV(3,Port_Data.Data_Transfer[189])OTL(Port_Data.Port_Read.[Port])OTL(Local_Control.4);
   42: XIC(Local_Control.5)XIO(Local_Control.6)EQU(K50ProTouch.Command,14)BTD(Port_Data.Data_Transfer[0],0,K50ProTouch.Write_Data.CC_Blue,0,8)BTD(Port_Data.Data_Transfer[1],0,K50ProTouch.Write_Data.CC2_Green,0,8)BTD(Port_Data.Data_Transfer[2],0,K50ProTouch.Write_Data.CC2_Red,0,8)OTU(Port_Data.Port_Read.[Port])OTL(Local_Control.6);
   43: NOP();
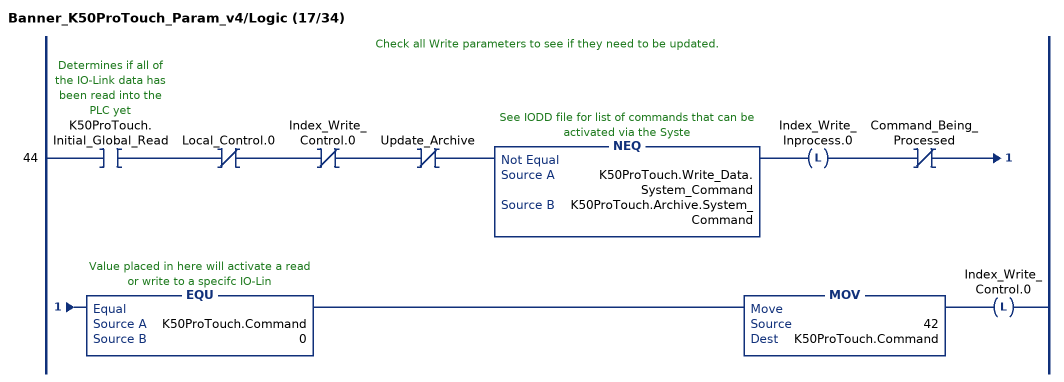
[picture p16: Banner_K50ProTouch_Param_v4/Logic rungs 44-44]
   // Check all Write parameters to see if they need to be updated.
   44: XIC(K50ProTouch.Initial_Global_Read)XIO(Local_Control.0)XIO(Index_Write_Control.0)XIO(Update_Archive)NEQ(K50ProTouch.Write_Data.System_Command,K50ProTouch.Archive.System_Command)OTL(Index_Write_Inprocess.0)XIO(Command_Being_Processed)EQU(K50ProTouch.Command,0)MOV(42,K50ProTouch.Command)OTL(Index_Write_Control.0);
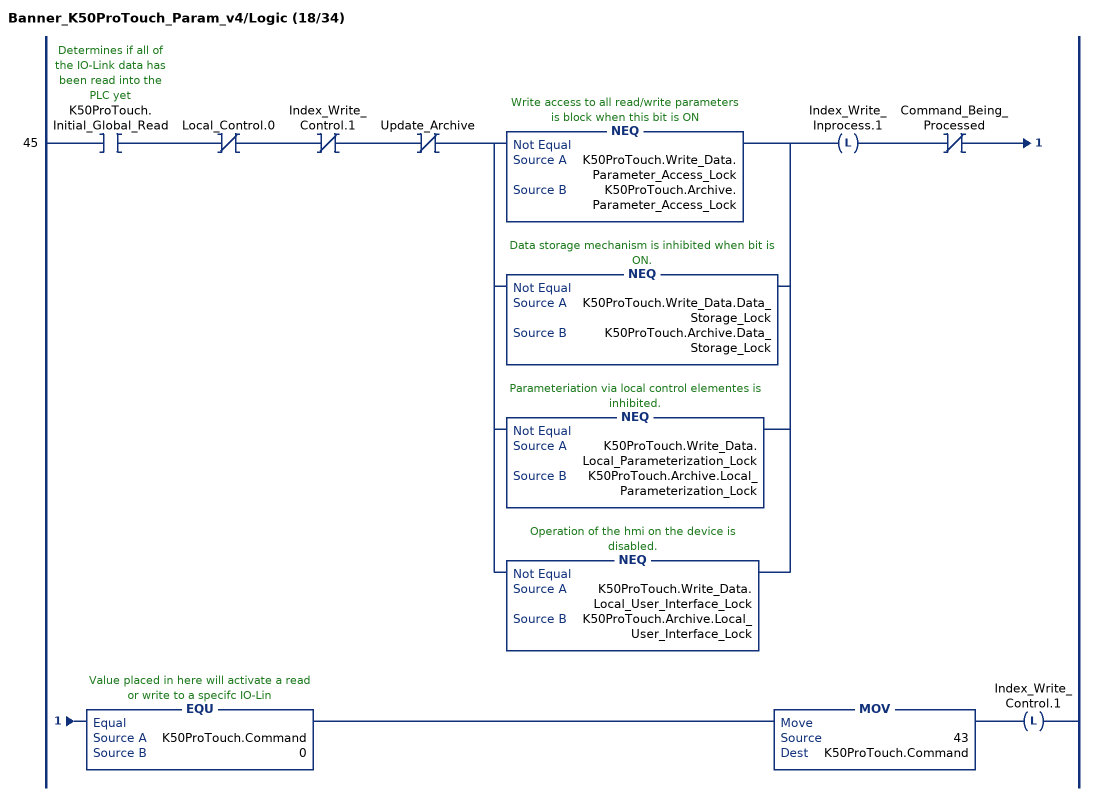
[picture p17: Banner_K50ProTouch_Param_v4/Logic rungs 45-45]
   45: XIC(K50ProTouch.Initial_Global_Read)XIO(Local_Control.0)XIO(Index_Write_Control.1)XIO(Update_Archive)[NEQ(K50ProTouch.Write_Data.Parameter_Access_Lock,K50ProTouch.Archive.Parameter_Access_Lock) ,NEQ(K50ProTouch.Write_Data.Data_Storage_Lock,K50ProTouch.Archive.Data_Storage_Lock) ,NEQ(K50ProTouch.Write_Data.Local_Parameterization_Lock,K50ProTouch.Archive.Local_Parameterization_Lock) ,NEQ(K50ProTouch.Write_Data.Local_User_Interface_Lock,K50ProTouch.Archive.Local_User_Interface_Lock) ]OTL(Index_Write_Inprocess.1)XIO(Command_Being_Processed)EQU(K50ProTouch.Command,0)MOV(43,K50ProTouch.Command)OTL(Index_Write_Control.1);
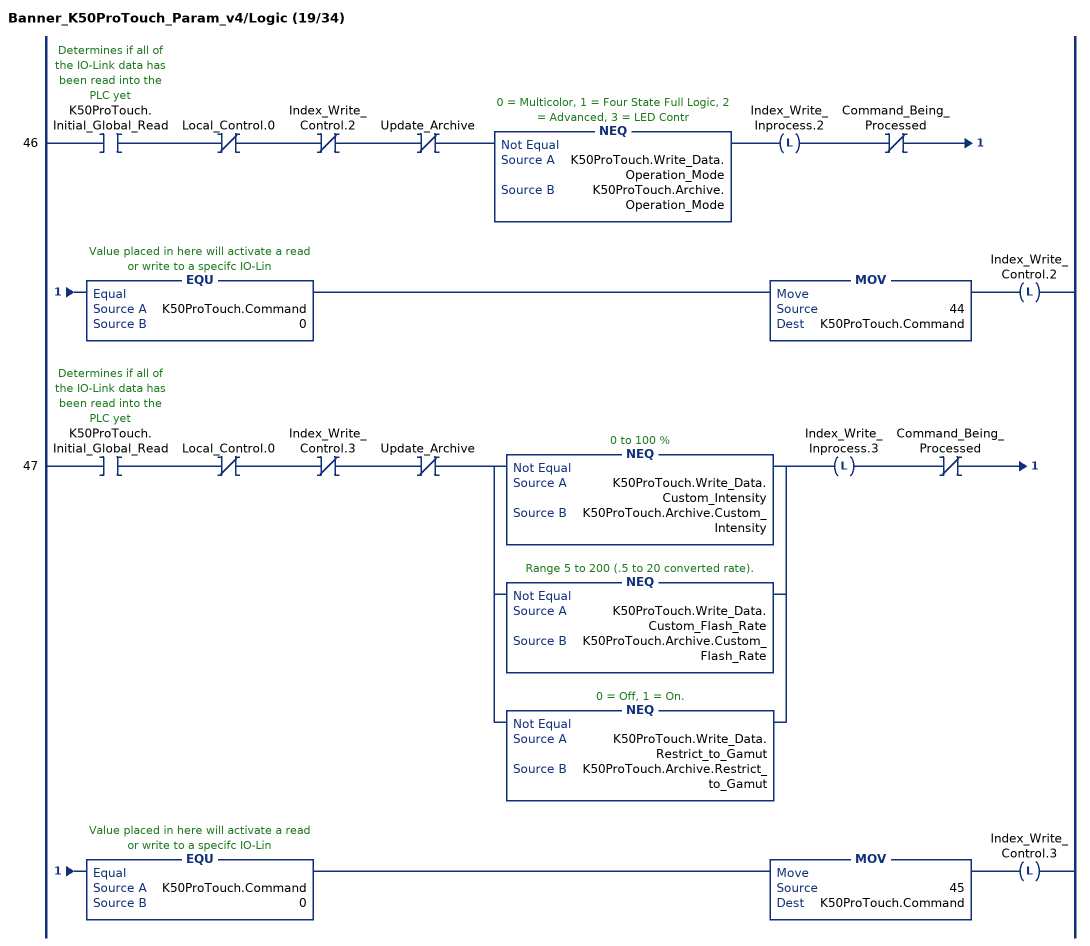
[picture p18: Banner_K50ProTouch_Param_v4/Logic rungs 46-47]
   46: XIC(K50ProTouch.Initial_Global_Read)XIO(Local_Control.0)XIO(Index_Write_Control.2)XIO(Update_Archive)NEQ(K50ProTouch.Write_Data.Operation_Mode,K50ProTouch.Archive.Operation_Mode)OTL(Index_Write_Inprocess.2)XIO(Command_Being_Processed)EQU(K50ProTouch.Command,0)MOV(44,K50ProTouch.Command)OTL(Index_Write_Control.2);
   47: XIC(K50ProTouch.Initial_Global_Read)XIO(Local_Control.0)XIO(Index_Write_Control.3)XIO(Update_Archive)[NEQ(K50ProTouch.Write_Data.Custom_Intensity,K50ProTouch.Archive.Custom_Intensity) ,NEQ(K50ProTouch.Write_Data.Custom_Flash_Rate,K50ProTouch.Archive.Custom_Flash_Rate) ,NEQ(K50ProTouch.Write_Data.Restrict_to_Gamut,K50ProTouch.Archive.Restrict_to_Gamut) ]OTL(Index_Write_Inprocess.3)XIO(Command_Being_Processed)EQU(K50ProTouch.Command,0)MOV(45,K50ProTouch.Command)OTL(Index_Write_Control.3);
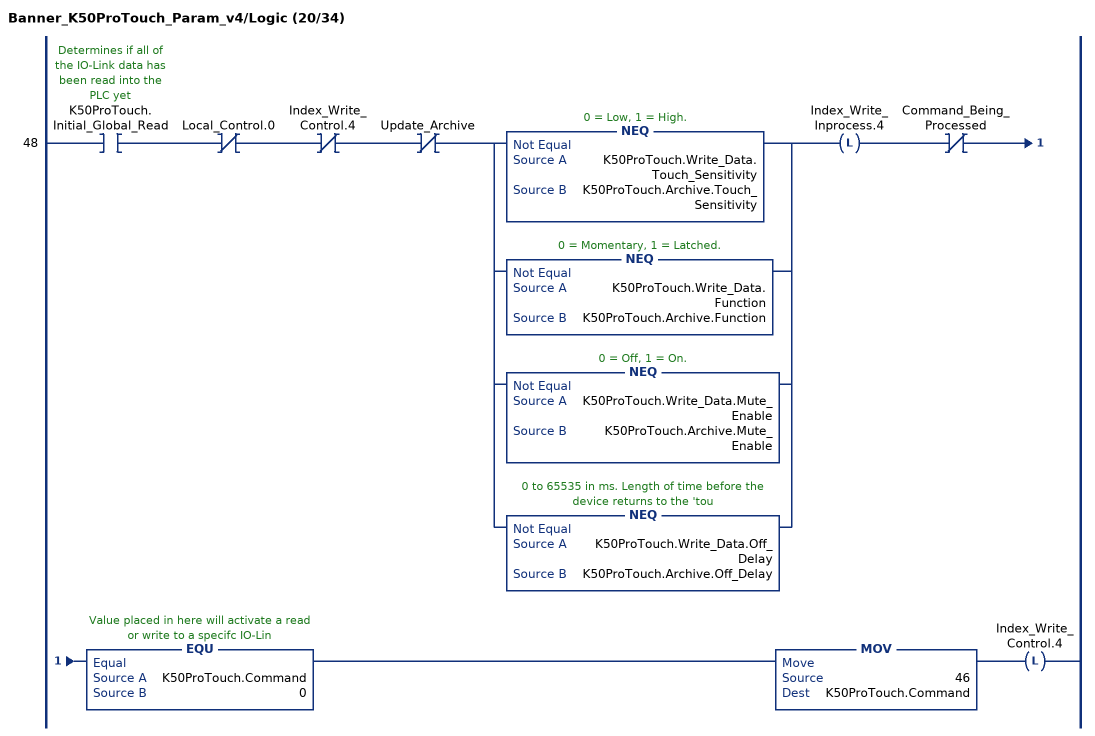
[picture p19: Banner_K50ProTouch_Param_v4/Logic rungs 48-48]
   48: XIC(K50ProTouch.Initial_Global_Read)XIO(Local_Control.0)XIO(Index_Write_Control.4)XIO(Update_Archive)[NEQ(K50ProTouch.Write_Data.Touch_Sensitivity,K50ProTouch.Archive.Touch_Sensitivity) ,NEQ(K50ProTouch.Write_Data.Function,K50ProTouch.Archive.Function) ,NEQ(K50ProTouch.Write_Data.Mute_Enable,K50ProTouch.Archive.Mute_Enable) ,NEQ(K50ProTouch.Write_Data.Off_Delay,K50ProTouch.Archive.Off_Delay) ]OTL(Index_Write_Inprocess.4)XIO(Command_Being_Processed)EQU(K50ProTouch.Command,0)MOV(46,K50ProTouch.Command)OTL(Index_Write_Control.4);
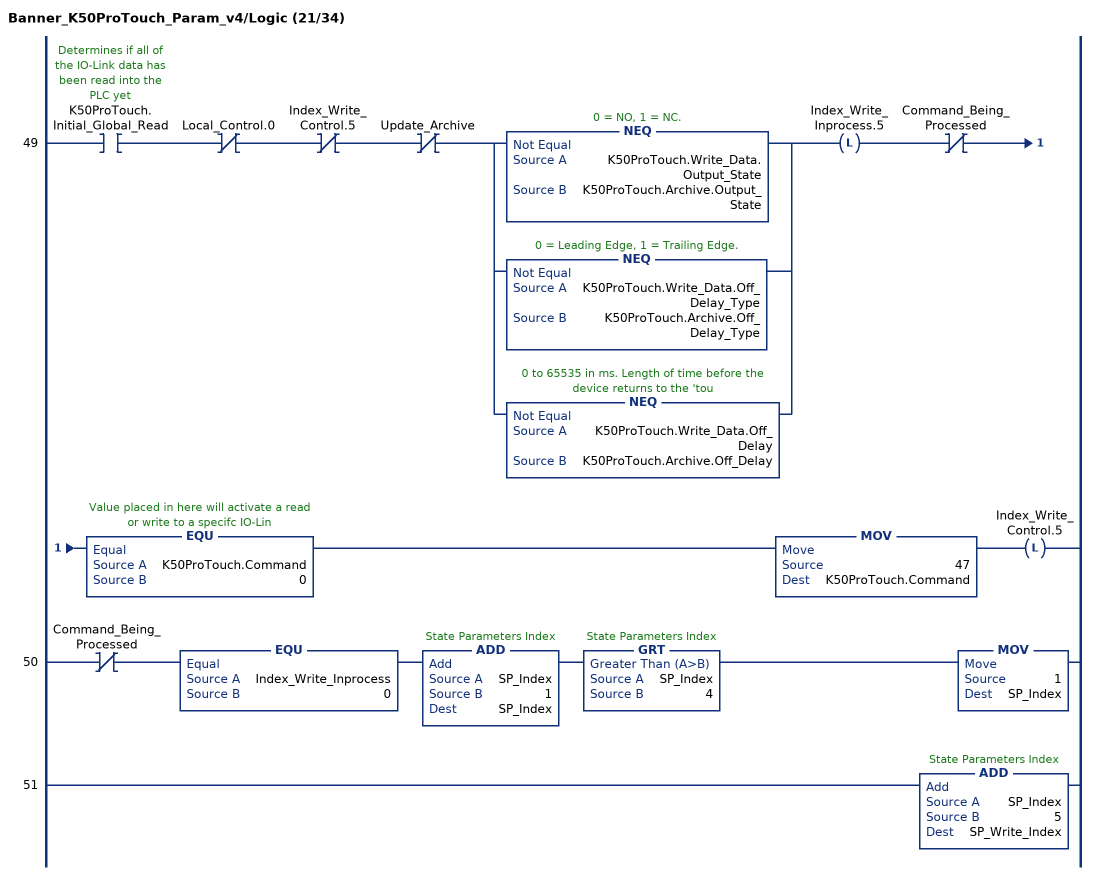
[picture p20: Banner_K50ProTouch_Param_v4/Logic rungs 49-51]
   49: XIC(K50ProTouch.Initial_Global_Read)XIO(Local_Control.0)XIO(Index_Write_Control.5)XIO(Update_Archive)[NEQ(K50ProTouch.Write_Data.Output_State,K50ProTouch.Archive.Output_State) ,NEQ(K50ProTouch.Write_Data.Off_Delay_Type,K50ProTouch.Archive.Off_Delay_Type) ,NEQ(K50ProTouch.Write_Data.Off_Delay,K50ProTouch.Archive.Off_Delay) ]OTL(Index_Write_Inprocess.5)XIO(Command_Being_Processed)EQU(K50ProTouch.Command,0)MOV(47,K50ProTouch.Command)OTL(Index_Write_Control.5);
   50: XIO(Command_Being_Processed)EQU(Index_Write_Inprocess,0)ADD(SP_Index,1,SP_Index)GRT(SP_Index,4)MOV(1,SP_Index);
   51: ADD(SP_Index,5,SP_Write_Index);
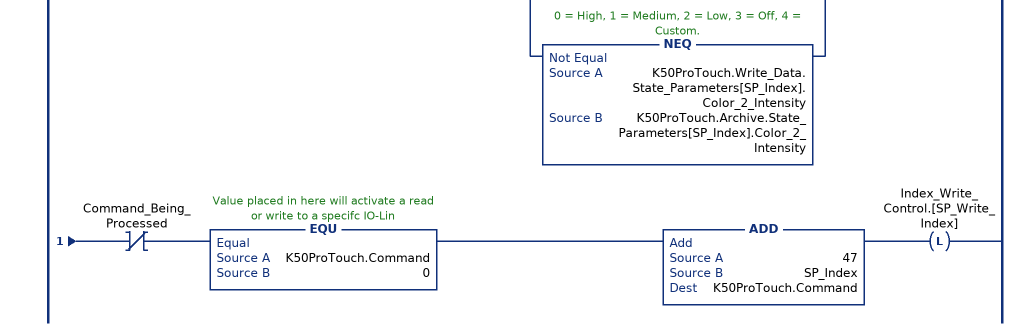
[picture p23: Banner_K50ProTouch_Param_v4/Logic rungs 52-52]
   52: XIC(K50ProTouch.Initial_Global_Read)XIO(Local_Control.0)XIO(Index_Write_Control.[SP_Write_Index])XIO(Update_Archive)[NEQ(K50ProTouch.Write_Data.State_Parameters[SP_Index].Type,K50ProTouch.Archive.State_Parameters[SP_Index].Type) ,NEQ(K50ProTouch.Write_Data.State_Parameters[SP_Index].Direction,K50ProTouch.Archive.State_Parameters[SP_Index].Direction) ,NEQ(K50ProTouch.Write_Data.State_Parameters[SP_Index].Pattern,K50ProTouch.Archive.State_Parameters[SP_Index].Pattern) ,NEQ(K50ProTouch.Write_Data.State_Parameters[SP_Index].Speed,K50ProTouch.Archive.State_Parameters[SP_Index].Speed) ,NEQ(K50ProTouch.Write_Data.State_Parameters[SP_Index].Vibration_Feedback,K50ProTouch.Archive.State_Parameters[SP_Index].Vibration_Feedback) ,NEQ(K50ProTouch.Write_Data.State_Parameters[SP_Index].Off_Delay_Type,K50ProTouch.Archive.State_Parameters[SP_Index].Off_Delay_Type) ,NEQ(K50ProTouch.Write_Data.State_Parameters[SP_Index].Off_Delay,K50ProTouch.Archive.State_Parameters[SP_Index].Off_Delay) ,NEQ(K50ProTouch.Write_Data.State_Parameters[SP_Index].Static_Sequence,K50ProTouch.Archive.State_Parameters[SP_Index].Static_Sequence) ,NEQ(K50ProTouch.Write_Data.State_Parameters[SP_Index].Sequence_Start_Location,K50ProTouch.Archive.State_Parameters[SP_Index].Sequence_Start_Location) ,NEQ(K50ProTouch.Write_Data.State_Parameters[SP_Index].Color_1,K50ProTouch.Archive.State_Parameters[SP_Index].Color_1) ,NEQ(K50ProTouch.Write_Data.State_Parameters[SP_Index].Color_1_Intensity,K50ProTouch.Archive.State_Parameters[SP_Index].Color_1_Intensity) ,NEQ(K50ProTouch.Write_Data.State_Parameters[SP_Index].Color_2,K50ProTouch.Archive.State_Parameters[SP_Index].Color_2) ,NEQ(K50ProTouch.Write_Data.State_Parameters[SP_Index].Color_2_Intensity,K50ProTouch.Archive.State_Parameters[SP_Index].Color_2_Intensity) ]OTL(Index_Write_Inprocess.[SP_Write_Index])XIO(Command_Being_Processed)EQU(K50ProTouch.Command,0)ADD(47,SP_Index,K50ProTouch.Command)OTL(Index_Write_Control.[SP_Write_Index]);
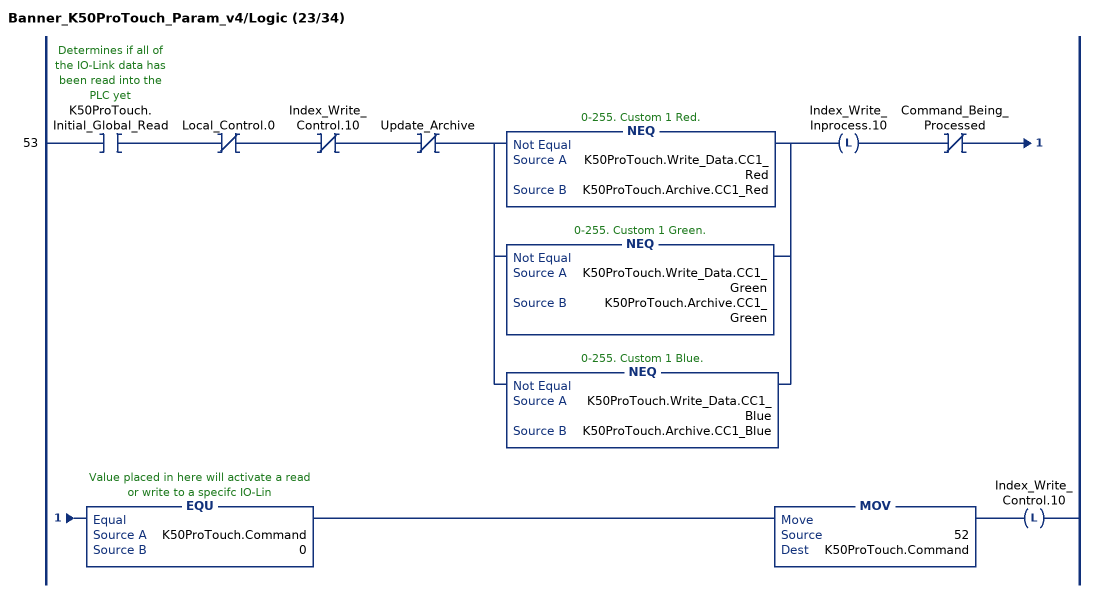
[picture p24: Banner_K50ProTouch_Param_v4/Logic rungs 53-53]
   53: XIC(K50ProTouch.Initial_Global_Read)XIO(Local_Control.0)XIO(Index_Write_Control.10)XIO(Update_Archive)[NEQ(K50ProTouch.Write_Data.CC1_Red,K50ProTouch.Archive.CC1_Red) ,NEQ(K50ProTouch.Write_Data.CC1_Green,K50ProTouch.Archive.CC1_Green) ,NEQ(K50ProTouch.Write_Data.CC1_Blue,K50ProTouch.Archive.CC1_Blue) ]OTL(Index_Write_Inprocess.10)XIO(Command_Being_Processed)EQU(K50ProTouch.Command,0)MOV(52,K50ProTouch.Command)OTL(Index_Write_Control.10);
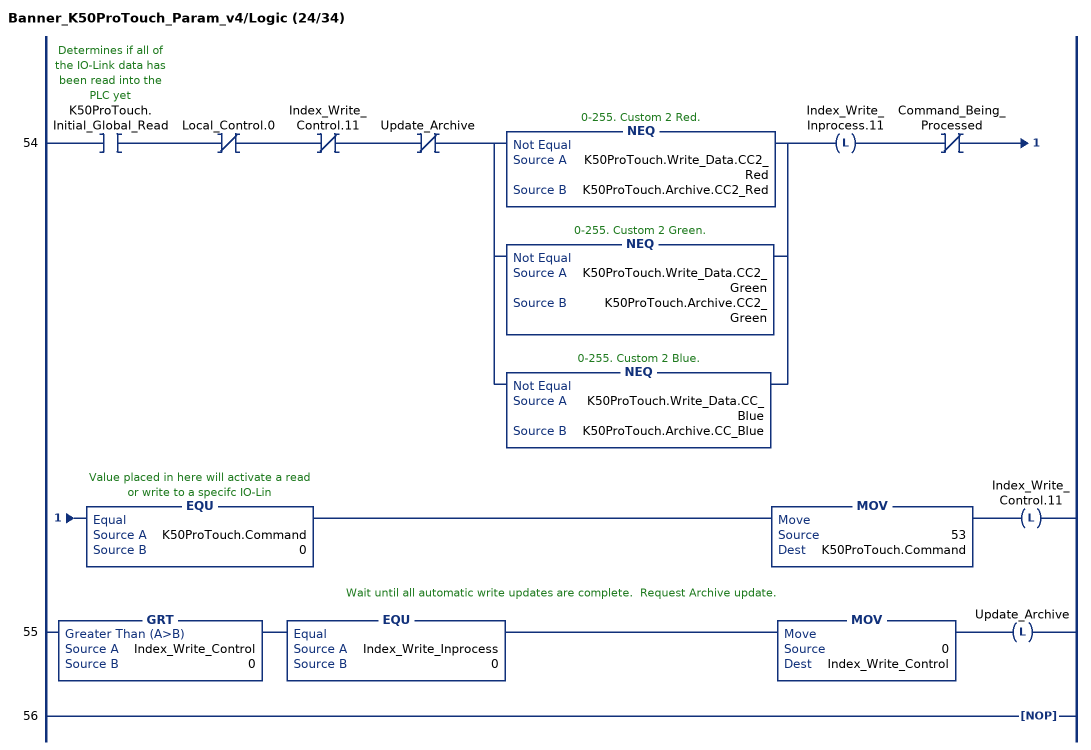
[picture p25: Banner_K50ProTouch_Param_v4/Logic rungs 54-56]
   54: XIC(K50ProTouch.Initial_Global_Read)XIO(Local_Control.0)XIO(Index_Write_Control.11)XIO(Update_Archive)[NEQ(K50ProTouch.Write_Data.CC2_Red,K50ProTouch.Archive.CC2_Red) ,NEQ(K50ProTouch.Write_Data.CC2_Green,K50ProTouch.Archive.CC2_Green) ,NEQ(K50ProTouch.Write_Data.CC_Blue,K50ProTouch.Archive.CC_Blue) ]OTL(Index_Write_Inprocess.11)XIO(Command_Being_Processed)EQU(K50ProTouch.Command,0)MOV(53,K50ProTouch.Command)OTL(Index_Write_Control.11);
   // Wait until all automatic write updates are complete.  Request Archive update.
   55: GRT(Index_Write_Control,0)EQU(Index_Write_Inprocess,0)MOV(0,Index_Write_Control)OTL(Update_Archive);
   56: NOP();
